//{{V2}}
ORGANIZATION_BLOCK OB35
TITLE= "Cyclic Interrupt"


AUTHOR:nb
FAMILY:nb
NAME:nb
VERSION:00.01


VAR_TEMP
       OB35_EV_CLASS:BYTE //Bits 0-3 = 1 (Coming event), Bits 4-7 = 1 (Event class 1)
       OB35_STRT_INF:BYTE //16#36 (OB 35 has started)
       OB35_PRIORITY:BYTE //Priority of OB Execution
       OB35_OB_NUMBR:BYTE //35 (Organization block 35, OB35)
       OB35_RESERVED_1:BYTE //Reserved for system
       OB35_RESERVED_2:BYTE //Reserved for system
       OB35_PHASE_OFFSET:WORD //Phase offset (msec)
       OB35_RESERVED_3:INT //Reserved for system
       OB35_EXC_FREQ:INT //Frequency of execution (msec)
       OB35_DATE_TIME:DATE_AND_TIME //Date and time OB35 started
END_VAR
BEGIN

END_ORGANIZATION_BLOCK
